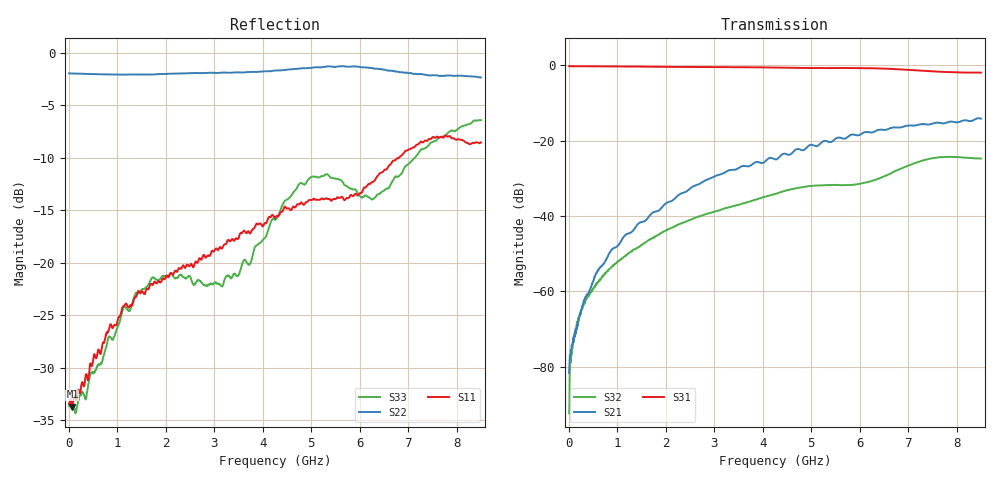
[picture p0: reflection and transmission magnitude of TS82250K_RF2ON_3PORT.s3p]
!Created with skrf (http://scikit-rf.org).
# GHz S RI R 50.0
!freq ReS11 ImS11 ReS12 ImS12 ReS13 ImS13
! ReS21 ImS21 ReS22 ImS22 ReS23 ImS23
! ReS31 ImS31 ReS32 ImS32 ReS33 ImS33
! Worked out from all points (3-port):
!   1601 points, 10 MHz to 8.5 GHz, reference 50 ohm
!   strongest paths, dB at 10 MHz, 2.132 GHz, 4.255 GHz, 6.378 GHz, 8.5 GHz:
!     S31: -0.2, -0.4, -0.6, -0.8, -2.0
!     S21: -81.7, -36.0, -25.0, -17.2, -14.2
!     S32: -92.4, -43.1, -34.2, -30.2, -24.7
!   lowest |S11| = -33.7 dB at 78.98 MHz (marker M1), VSWR 1.04, Z = 52.1 + j0.185 ohm
!   |S11| at or under -10 dB: start of sweep to 6.817 GHz
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0.01  0.0213 -0.00039  6.98e-05 2.49e-05  0.9732 -0.00498
      6.28e-05 5.37e-05  -0.7962 0.00472  1.27e-05 5.26e-05
      0.9731 -0.00502  1.21e-05 2.08e-05  0.0206 0.00197
0.07898125  0.0205 0.00178  0.000111 0.000171  0.9712 -0.0261
            0.000105 0.000171  -0.7944 0.0333  7.45e-05 0.000172
            0.9712 -0.0261  5.04e-05 0.000167  0.0209 0.00188
0.3973563  0.0247 0.0124  -0.00031 0.000861  0.9611 -0.1271
           -0.000316 0.000846  -0.7736 0.1637  1.77e-05 0.000857
           0.961 -0.1267  1.73e-05 0.000855  0.0207 0.0151
1.166762  0.052 0.0362  -0.00348 0.00435  0.8945 -0.3565
          -0.00349 0.00433  -0.6413 0.4535  -0.000358 0.00292
          0.8943 -0.3565  -0.000338 0.00293  0.0287 0.0545
2.578225  0.0955 -0.00148  -0.0122 0.0217  0.6411 -0.7002
          -0.0122 0.0218  -0.224 0.767  0.000975 0.00925
          0.6392 -0.7011  0.00098 0.00923  0.0393 0.0678
3.4909  0.1232 -0.0398  -0.0072 0.0421  0.4062 -0.8516
        -0.00719 0.0422  0.0872 0.8  0.00477 0.0132
        0.402 -0.8531  0.00474 0.0131  0.0428 0.0753
4.255  0.1353 -0.092  0.00497 0.0562  0.1836 -0.9156
       0.00505 0.0563  0.3622 0.7365  0.0102 0.0167
       0.1767 -0.9162  0.0102 0.0167  0.0807 0.1383
5.013794  0.0838 -0.1802  0.0246 0.0847  -0.0347 -0.9185
          0.0246 0.0846  0.5766 0.6209  0.0191 0.0163
          -0.0444 -0.9178  0.0191 0.0162  0.1448 0.2122
6.75955  -0.2881 -0.1192  0.1168 0.0932  -0.5306 -0.7114
         0.1167 0.0934  0.7579 0.2882  0.034 0.0213
         -0.5447 -0.6992  0.0341 0.0212  0.05 0.2525
8.5  -0.3719 0.0365  0.1953 -0.0183  -0.7663 -0.2282
     0.1949 -0.018  0.7186 -0.2521  0.0525 -0.0242
     -0.7652 -0.2291  0.0525 -0.0243  0.4267 0.2132
